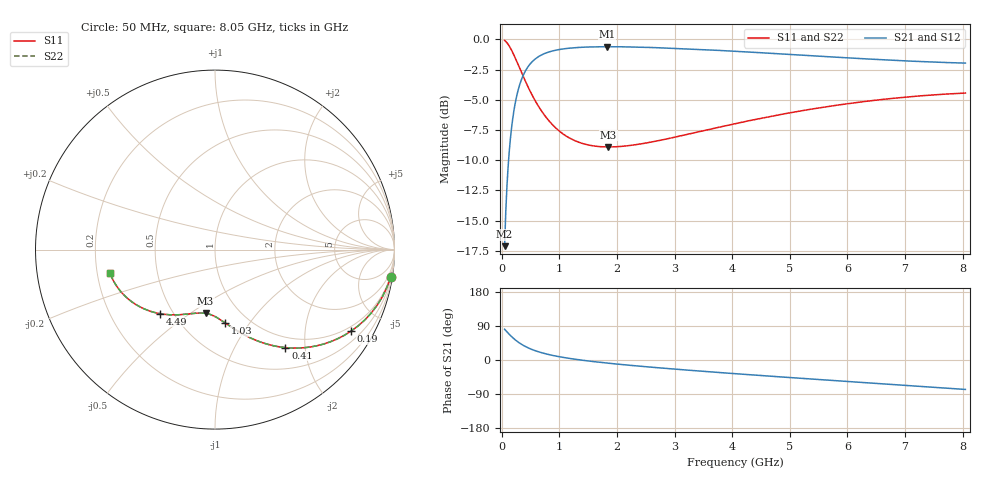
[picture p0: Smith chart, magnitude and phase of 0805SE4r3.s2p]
! AVX Thin Film Operation		Date: August 2001
! Description: Accu-P® Series, Thin Film, SMD, RF Capacitor
! Part Number: 08051J4R3ABT
! 50 MHz  -  8.05 GHz
! Serial Measurements
# mhz S db R 50
!	S11		S21		S12		S22
!	dB	Phase	dB	Phase	dB	Phase	dB	Phase
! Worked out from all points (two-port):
!   401 points, 50 MHz to 8.05 GHz, reference 50 ohm
!   highest |S21| = -0.60 dB at 1.83 GHz (marker M1); lowest = -17.1 dB at 50 MHz (marker M2)
!   |S21| within 3 dB of the highest: 322.1 MHz to end of sweep
!   lowest |S11| = -8.9 dB at 1.85 GHz (marker M3), VSWR 2.12, Z = 35.3 - j28.8 ohm
!   |S11| at or under -10 dB: nowhere
!   |S22| runs from -8.9 to -0.1 dB; largest |S21 - S12| = 0
!   S11 on the Smith chart (normalised r, x): 50 MHz: 1, -13; 190 MHz: 0.83, -3.43; 410 MHz: 0.82, -1.64; 1.03 GHz: 0.79, -0.77; 4.49 GHz: 0.42, -0.39; 8.05 GHz: 0.25, -0.10
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50  -0.09 -8.8  -17.12 81.2  -17.12 81.2  -0.09 -8.8
90  -0.27 -15.6  -12.21 74.4  -12.21 74.4  -0.27 -15.6
110  -0.40 -18.9  -10.60 71.1  -10.60 71.1  -0.40 -18.9
130  -0.54 -22.1  -9.31 67.9  -9.31 67.9  -0.54 -22.1
190  -1.07 -31.0  -6.59 59.0  -6.59 59.0  -1.07 -31.0
230  -1.48 -36.2  -5.39 53.8  -5.39 53.8  -1.48 -36.2
290  -2.14 -43.2  -4.11 46.8  -4.11 46.8  -2.14 -43.2
410  -3.45 -54.3  -2.62 35.7  -2.62 35.7  -3.45 -54.3
530  -4.63 -62.5  -1.84 27.4  -1.84 27.4  -4.63 -62.5
670  -5.78 -69.8  -1.34 20.2  -1.34 20.2  -5.78 -69.8
830  -6.80 -76.1  -1.02 13.9  -1.02 13.9  -6.80 -76.1
1030  -7.70 -82.1  -0.81 7.8  -0.81 7.8  -7.70 -82.1
1390  -8.60 -90.3  -0.65 -0.4  -0.65 -0.4  -8.60 -90.3
1830  -8.90 -98.0  -0.60 -8.1  -0.60 -8.1  -8.90 -98.1
1850  -8.90 -98.4  -0.60 -8.4  -0.60 -8.4  -8.90 -98.4
2730  -8.37 -110.6  -0.69 -20.7  -0.69 -20.7  -8.37 -110.6
3370  -7.70 -118.3  -0.81 -28.4  -0.81 -28.4  -7.70 -118.3
4050  -6.98 -126.0  -0.98 -36.1  -0.98 -36.1  -6.98 -126.0
4490  -6.54 -130.8  -1.10 -40.9  -1.10 -40.9  -6.54 -130.8
5390  -5.76 -140.2  -1.35 -50.4  -1.35 -50.4  -5.76 -140.2
6730  -4.91 -154.0  -1.71 -64.1  -1.71 -64.1  -4.91 -154.0
8050  -4.44 -167.5  -1.96 -77.7  -1.96 -77.7  -4.44 -167.5
